(* Logix 5000 AddOnInstructionDefinition export SIKO_AG2X; software revision 18.02 *)

ADD_ON_INSTRUCTION SIKO_AG2X   (* revision 1.6, vendor SIKO GmbH *)
// SIKO DriveLine AG2X AOI
// Revision note:
// minor changes, timeout feature added
VAR_INPUT
   Cmd_OFF1 : BOOL; {visible}
   Cmd_OFF2 : BOOL; {visible}
   Cmd_OFF3 : BOOL; {visible}
   Cmd_Intermediate_stop : BOOL; {visible}
   Cmd_Start_travel_job : BOOL; {visible}
   Cmd_Acknowledge_error : BOOL; {visible}
   Cmd_Inching_mode_1 : BOOL; {visible}
   Cmd_Inching_2_Pos : BOOL; {visible}
   Cmd_Inching_2_Neg : BOOL; {visible}
   Cmd_Move_relative : BOOL; {visible}
END_VAR
VAR_IN_OUT
   DC_OUTPUT : SINT[7]; {required}
   DC_INPUT : SINT[7]; {required}
END_VAR
VAR_INPUT
   Cmd_Start_read : BOOL; {visible}
   Cmd_Start_write : BOOL; {visible}
END_VAR
VAR_IN_OUT
   GetMsg : MESSAGE; {required}
   GetMsgData : SINT[4]; {required}
   SetMsg : MESSAGE; {required}
   SetMsgData : SINT[4]; {required}
END_VAR
VAR_OUTPUT
   count_read : INT; {access Read Only, visible}
   read_error : DINT; {access Read Only, visible}
   count_write : INT; {access Read Only, visible}
   write_error : DINT; {access Read Only, visible}
END_VAR
VAR_INPUT
   Cmd_DO1 : BOOL; {visible}
END_VAR
VAR_OUTPUT
   ACTUAL_VALUE : DINT; {access Read Only, visible}
END_VAR
VAR_INPUT
   TARGET_VALUE : DINT; {visible}
   Cmd_Copy_r_to_w : BOOL; {visible}
   Cmd_BIT9 : BOOL;
   Cmd_BIT10 : BOOL;
   Cmd_BIT11 : BOOL;
   Cmd_BIT12 : BOOL;
   Cmd_BIT13 : BOOL;
   Cmd_BIT14 : BOOL;
   Cmd_BIT15 : BOOL;
END_VAR
VAR_OUTPUT
   i0513_Led_functionality_r : SINT; {access Read Only}
END_VAR
VAR_INPUT
   i0513_Led_functionality_w : SINT;
END_VAR
VAR_OUTPUT
   i0545_Si_baudrate_r : SINT; {access Read Only}
END_VAR
VAR_INPUT
   i0545_Si_baudrate_w : SINT := 1;
END_VAR
VAR_OUTPUT
   i0769_DO_1_functionality_r : SINT; {access Read Only}
END_VAR
VAR_INPUT
   i0769_DO_1_functionality_w : SINT;
END_VAR
VAR_OUTPUT
   i0770_DO_functionalities_state_r : DINT; {access Read Only}
   i0771_DO_polarity_r : SINT; {access Read Only}
END_VAR
VAR_INPUT
   i0771_DO_polarity_w : SINT;
END_VAR
VAR_OUTPUT
   i1025_DI_1_functionality_r : SINT; {access Read Only}
END_VAR
VAR_INPUT
   i1025_DI_1_functionality_w : SINT;
END_VAR
VAR_OUTPUT
   i1026_DI_2_functionality_r : SINT; {access Read Only}
END_VAR
VAR_INPUT
   i1026_DI_2_functionality_w : SINT;
END_VAR
VAR_OUTPUT
   i1027_DI_3_functionality_r : SINT; {access Read Only}
END_VAR
VAR_INPUT
   i1027_DI_3_functionality_w : SINT;
END_VAR
VAR_OUTPUT
   i1028_DI_4_functionality_r : SINT; {access Read Only}
END_VAR
VAR_INPUT
   i1028_DI_4_functionality_w : SINT;
END_VAR
VAR_OUTPUT
   i1029_DI_functionalities_state_r : DINT; {access Read Only}
   i1030_DI_polarity_r : SINT; {access Read Only}
END_VAR
VAR_INPUT
   i1030_DI_polarity_w : SINT;
END_VAR
VAR_OUTPUT
   i1537_Controller_parameter_P_r : INT; {access Read Only}
END_VAR
VAR_INPUT
   i1537_Controller_parameter_P_w : INT := 300;
END_VAR
VAR_OUTPUT
   i1538_Controller_parameter_I_r : INT; {access Read Only}
END_VAR
VAR_INPUT
   i1538_Controller_parameter_I_w : INT := 2;
END_VAR
VAR_OUTPUT
   i1539_Controller_parameter_D_r : INT; {access Read Only}
END_VAR
VAR_INPUT
   i1539_Controller_parameter_D_w : INT;
END_VAR
VAR_OUTPUT
   i1540_a_Pos_r : INT; {access Read Only}
END_VAR
VAR_INPUT
   i1540_a_Pos_w : INT := 50;
END_VAR
VAR_OUTPUT
   i1541_v_Pos_r : INT; {access Read Only}
END_VAR
VAR_INPUT
   i1541_v_Pos_w : INT := 10;
END_VAR
VAR_OUTPUT
   i1542_d_Pos_r : INT; {access Read Only}
END_VAR
VAR_INPUT
   i1542_d_Pos_w : INT := 101;
END_VAR
VAR_OUTPUT
   i1543_a_Rot_r : INT; {access Read Only}
END_VAR
VAR_INPUT
   i1543_a_Rot_w : INT := 50;
END_VAR
VAR_OUTPUT
   i1544_a_Inch_r : INT; {access Read Only}
END_VAR
VAR_INPUT
   i1544_a_Inch_w : INT := 50;
END_VAR
VAR_OUTPUT
   i1545_v_Inch_r : INT; {access Read Only}
END_VAR
VAR_INPUT
   i1545_v_Inch_w : INT := 10;
END_VAR
VAR_OUTPUT
   i1546_Pos_window_r : INT; {access Read Only}
END_VAR
VAR_INPUT
   i1546_Pos_window_w : INT := 10;
END_VAR
VAR_OUTPUT
   i1547_Gear_ratio_numerator_r : INT; {access Read Only}
END_VAR
VAR_INPUT
   i1547_Gear_ratio_numerator_w : INT := 1;
END_VAR
VAR_OUTPUT
   i1548_Gear_ratio_denominator_r : INT; {access Read Only}
END_VAR
VAR_INPUT
   i1548_Gear_ratio_denominator_w : INT := 1;
END_VAR
VAR_OUTPUT
   i1549_Spindle_pitch_r : DINT; {access Read Only}
END_VAR
VAR_INPUT
   i1549_Spindle_pitch_w : DINT;
END_VAR
VAR_OUTPUT
   i1550_Calibration_value_r : DINT; {access Read Only}
END_VAR
VAR_INPUT
   i1550_Calibration_value_w : DINT;
END_VAR
VAR_OUTPUT
   i1551_Limit_1_r : DINT; {access Read Only}
END_VAR
VAR_INPUT
   i1551_Limit_1_w : DINT := 99999;
END_VAR
VAR_OUTPUT
   i1552_Limit_2_r : DINT; {access Read Only}
END_VAR
VAR_INPUT
   i1552_Limit_2_w : DINT := -19999;
END_VAR
VAR_OUTPUT
   i1553_Delta_inch_r : DINT; {access Read Only}
END_VAR
VAR_INPUT
   i1553_Delta_inch_w : DINT := 720;
END_VAR
VAR_OUTPUT
   i1554_Sense_of_rotation_r : SINT; {access Read Only}
END_VAR
VAR_INPUT
   i1554_Sense_of_rotation_w : SINT;
END_VAR
VAR_OUTPUT
   i1555_Pos_type_r : SINT; {access Read Only}
END_VAR
VAR_INPUT
   i1555_Pos_type_w : SINT;
END_VAR
VAR_OUTPUT
   i1556_Operating_mode_r : SINT; {access Read Only}
END_VAR
VAR_INPUT
   i1556_Operating_mode_w : SINT;
END_VAR
VAR_OUTPUT
   i1557_Inching_2_stop_mode_r : SINT; {access Read Only}
END_VAR
VAR_INPUT
   i1557_Inching_2_stop_mode_w : SINT;
END_VAR
VAR_OUTPUT
   i1558_Inpos_mode_r : SINT; {access Read Only}
END_VAR
VAR_INPUT
   i1558_Inpos_mode_w : SINT;
END_VAR
VAR_OUTPUT
   i1559_Loop_length_r : INT;
END_VAR
VAR_INPUT
   i1559_Loop_length_w : INT := 360;
END_VAR
VAR_OUTPUT
   i1560_Contouring_error_limit_r : INT; {access Read Only}
END_VAR
VAR_INPUT
   i1560_Contouring_error_limit_w : INT := 400;
END_VAR
VAR_OUTPUT
   i1561_Current_limiting_r : SINT; {access Read Only}
END_VAR
VAR_INPUT
   i1561_Current_limiting_w : SINT := 110;
END_VAR
VAR_OUTPUT
   i1562_Inching_2_Offset_r : SINT; {access Read Only}
END_VAR
VAR_INPUT
   i1562_Inching_2_Offset_w : SINT := 100;
END_VAR
VAR_OUTPUT
   i1563_Inching_2_acceleration_type_r : SINT; {access Read Only}
END_VAR
VAR_INPUT
   i1563_Inching_2_acceleration_type_w : SINT;
END_VAR
VAR_OUTPUT
   i1564_Offset_r : DINT; {access Read Only}
END_VAR
VAR_INPUT
   i1564_Offset_w : DINT;
END_VAR
VAR_OUTPUT
   i2338_Pcm_pos_1_r : DINT; {access Read Only}
END_VAR
VAR_INPUT
   i2338_Pcm_pos_1_w : DINT; {access Read Only}
END_VAR
VAR_OUTPUT
   i2339_Pcm_pos_2_r : DINT; {access Read Only}
END_VAR
VAR_INPUT
   i2339_Pcm_pos_2_w : DINT; {access Read Only}
END_VAR
VAR_OUTPUT
   i2340_Pcm_pos_3_r : DINT; {access Read Only}
END_VAR
VAR_INPUT
   i2340_Pcm_pos_3_w : DINT; {access Read Only}
END_VAR
VAR_OUTPUT
   i2341_Pcm_pos_4_r : DINT; {access Read Only}
END_VAR
VAR_INPUT
   i2341_Pcm_pos_4_w : DINT; {access Read Only}
END_VAR
VAR_OUTPUT
   i2342_Pcm_pos_5_r : DINT; {access Read Only}
END_VAR
VAR_INPUT
   i2342_Pcm_pos_5_w : DINT; {access Read Only}
END_VAR
VAR_OUTPUT
   i2343_Pcm_pos_6_r : DINT; {access Read Only}
END_VAR
VAR_INPUT
   i2343_Pcm_pos_6_w : DINT; {access Read Only}
END_VAR
VAR_OUTPUT
   i2344_Pcm_pos_7_r : DINT; {access Read Only}
END_VAR
VAR_INPUT
   i2344_Pcm_pos_7_w : DINT; {access Read Only}
END_VAR
VAR_OUTPUT
   i2370_Pcm_acc_1_r : INT; {access Read Only}
END_VAR
VAR_INPUT
   i2370_Pcm_acc_1_w : INT := 50; {access Read Only}
END_VAR
VAR_OUTPUT
   i2371_Pcm_acc_2_r : INT; {access Read Only}
END_VAR
VAR_INPUT
   i2371_Pcm_acc_2_w : INT := 50; {access Read Only}
END_VAR
VAR_OUTPUT
   i2372_Pcm_acc_3_r : INT; {access Read Only}
END_VAR
VAR_INPUT
   i2372_Pcm_acc_3_w : INT := 50; {access Read Only}
END_VAR
VAR_OUTPUT
   i2373_Pcm_acc_4_r : INT; {access Read Only}
END_VAR
VAR_INPUT
   i2373_Pcm_acc_4_w : INT := 50;
END_VAR
VAR_OUTPUT
   i2374_Pcm_acc_5_r : INT; {access Read Only}
END_VAR
VAR_INPUT
   i2374_Pcm_acc_5_w : INT := 50;
END_VAR
VAR_OUTPUT
   i2375_Pcm_acc_6_r : INT; {access Read Only}
END_VAR
VAR_INPUT
   i2375_Pcm_acc_6_w : INT := 50;
END_VAR
VAR_OUTPUT
   i2376_Pcm_acc_7_r : INT; {access Read Only}
END_VAR
VAR_INPUT
   i2376_Pcm_acc_7_w : INT := 50;
END_VAR
VAR_OUTPUT
   i2402_Pcm_vel_1_r : INT; {access Read Only}
END_VAR
VAR_INPUT
   i2402_Pcm_vel_1_w : INT := 10;
END_VAR
VAR_OUTPUT
   i2403_Pcm_vel_2_r : INT; {access Read Only}
END_VAR
VAR_INPUT
   i2403_Pcm_vel_2_w : INT := 10;
END_VAR
VAR_OUTPUT
   i2404_Pcm_vel_3_r : INT; {access Read Only}
END_VAR
VAR_INPUT
   i2404_Pcm_vel_3_w : INT := 10;
END_VAR
VAR_OUTPUT
   i2405_Pcm_vel_4_r : INT; {access Read Only}
END_VAR
VAR_INPUT
   i2405_Pcm_vel_4_w : INT := 10;
END_VAR
VAR_OUTPUT
   i2406_Pcm_vel_5_r : INT; {access Read Only}
END_VAR
VAR_INPUT
   i2406_Pcm_vel_5_w : INT := 10;
END_VAR
VAR_OUTPUT
   i2407_Pcm_vel_6_r : INT; {access Read Only}
END_VAR
VAR_INPUT
   i2407_Pcm_vel_6_w : INT := 10;
END_VAR
VAR_OUTPUT
   i2408_Pcm_vel_7_r : INT; {access Read Only}
END_VAR
VAR_INPUT
   i2408_Pcm_vel_7_w : INT := 10;
END_VAR
VAR_OUTPUT
   i2434_Pcm_dec_1_r : INT; {access Read Only}
END_VAR
VAR_INPUT
   i2434_Pcm_dec_1_w : INT := 101;
END_VAR
VAR_OUTPUT
   i2435_Pcm_dec_2_r : INT; {access Read Only}
END_VAR
VAR_INPUT
   i2435_Pcm_dec_2_w : INT := 101;
END_VAR
VAR_OUTPUT
   i2436_Pcm_dec_3_r : INT; {access Read Only}
END_VAR
VAR_INPUT
   i2436_Pcm_dec_3_w : INT := 101;
END_VAR
VAR_OUTPUT
   i2437_Pcm_dec_4_r : INT; {access Read Only}
END_VAR
VAR_INPUT
   i2437_Pcm_dec_4_w : INT := 101;
END_VAR
VAR_OUTPUT
   i2438_Pcm_dec_5_r : INT; {access Read Only}
END_VAR
VAR_INPUT
   i2438_Pcm_dec_5_w : INT := 101;
END_VAR
VAR_OUTPUT
   i2439_Pcm_dec_6_r : INT; {access Read Only}
END_VAR
VAR_INPUT
   i2439_Pcm_dec_6_w : INT := 101;
END_VAR
VAR_OUTPUT
   i2440_Pcm_dec_7_r : INT; {access Read Only}
END_VAR
VAR_INPUT
   i2440_Pcm_dec_7_w : INT := 101;
END_VAR
VAR_OUTPUT
   i2561_Output_stage_temperature_r : INT; {access Read Only}
   i2562_Voltage_of_control_r : INT; {access Read Only}
   i2563_Voltage_of_output_power_stage_r : INT; {access Read Only}
   i2564_Voltage_of_battery_r : INT; {access Read Only}
   i2565_Motor_Current_r : INT; {access Read Only}
   i2566_Actual_position_r : DINT; {access Read Only}
   i2567_Actual_rotational_speed_r : INT; {access Read Only}
   i2568_Serial_number_r : DINT; {access Read Only}
   i2569_Production_date_r : DINT; {access Read Only}
   i2570_Sw_motor_controller_r : DINT; {access Read Only}
   i2571_Gear_reduction_r : INT; {access Read Only}
   i2572_System_status_word_r : INT;
   i2573_Encoder_resolution_r : INT; {access Read Only}
   i2574_Device_id_r : SINT; {access Read Only}
   i2817_Number_of_errors_r : SINT; {access Read Only}
   i2818_Error_nbr_1_r : SINT; {access Read Only}
   i2819_Error_nbr_2_r : SINT; {access Read Only}
   i2820_Error_nbr_3_r : SINT; {access Read Only}
   i2821_Error_nbr_4_r : SINT; {access Read Only}
   i2822_Error_nbr_5_r : SINT; {access Read Only}
   i2823_Error_nbr_6_r : SINT; {access Read Only}
   i2824_Error_nbr_7_r : SINT; {access Read Only}
   i2825_Error_nbr_8_r : SINT; {access Read Only}
   i2826_Error_nbr_9_r : SINT; {access Read Only}
   i2827_Error_nbr_10_r : SINT; {access Read Only}
   i3073_S_command_r : SINT; {access Read Only}
END_VAR
VAR_INPUT
   i3073_S_command_w : SINT;
END_VAR
VAR_OUTPUT
   Sts_BIT13 : BOOL; {access Read Only}
   Sts_BIT14 : BOOL; {access Read Only}
   Sts_BIT15 : BOOL; {access Read Only}
   Sts_Supply : BOOL; {access Read Only, visible}
   Sts_Readiness_to_travel : BOOL; {access Read Only, visible}
   Sts_Upper_limit : BOOL; {access Read Only, visible}
   Sts_Lower_limit : BOOL; {access Read Only, visible}
   Sts_Actuator_travels_stands : BOOL; {access Read Only, visible}
   Sts_InPos : BOOL; {access Read Only, visible}
   Sts_Active_travel_job : BOOL; {access Read Only, visible}
   Sts_Error : BOOL; {access Read Only, visible}
   Sts_Operation_enabled : BOOL; {access Read Only, visible}
   Sts_Switch_lock : BOOL; {access Read Only, visible}
   Sts_Travel_job_acknowledge : BOOL; {access Read Only, visible}
   Sts_Battery_warning : BOOL; {access Read Only, visible}
   Sts_Current_limiting : BOOL; {access Read Only, visible}
   Sts_DI1 : BOOL; {access Read Only, visible}
   Sts_DI2 : BOOL; {access Read Only, visible}
   Sts_DI3 : BOOL; {access Read Only, visible}
   Sts_DI4 : BOOL; {access Read Only, visible}
   Sts_Done : BOOL; {access Read Only, visible}
   Sts_Busy : BOOL; {access Read Only, visible}
   Sts_General_error : BOOL; {access Read Only, visible}
END_VAR
VAR_INPUT
   Timeout : DINT := 5000; {visible}
END_VAR
VAR
   BTDT_01 : FBD_BIT_FIELD_DISTRIBUTE := (Length := 1); {access None}
   BTDT_02 : FBD_BIT_FIELD_DISTRIBUTE := (Length := 1); {access None}
   DC_INPUT_BUF : SINT[7]; {access None}
   DC_OUTPUT_BUF : SINT[7]; {access None}
   GetMsgStep : INT; {access None}
   SetMsgStep : INT; {access None}
   LD_OUT : DINT; {access None}
   OSR_copy : BOOL; {access None}
   OSR_read : BOOL; {access None}
   OSR_write : BOOL; {access None}
   SetMsgFlags : INT; {access None}
   GetMsgFlags : INT; {access None}
   COUNTER_WRITE : INT; {access None}
   COUNTER_READ : INT; {access None}
   COUNTER_COPY : INT; {access None}
   tTOutWrite : FBD_TIMER; {access None}
   tTOutRead : FBD_TIMER; {access None}
END_VAR

ROUTINE Logic   (* structured text *)
   ///////////////////////////////////////////////////////////////////////////////////////////////
   // Name:	SIKO_AG2X
   ///////////////////////////////////////////////////////////////////////////////////////////////
   // Version history
   ///////////////////////////////////////////////////////////////////////////////////////////////
   // Date        | Version  | created under          	| Author    		| Remark
   // dd.mm.yyyy  | 		  |							|					|
   // -----------------------------------------------------------------------------------
   // 17.06.2014  | 1.0.0    | V20.01.00 (CPR 9 SR 5) 	| SIKO GmbH / hof 	| first release
   // 04.07.2014  | 1.1.0	  | V20.01.00 (CPR 9 SR 5)  | SIKO GmbH / hof 	| synchronous access
   // 06.10.2014  | 1.2.0    | V20.01.00 (CPR 9 SR 5)  | SIKO GmbH / hof 	| minor changes
   // 04.02.2015  | 1.3.0    | V20.01.00 (CPR 9 SR 5)  | SIKO GmbH / hof   | signature protection
   // 05.03.2015  | 1.4.0    | V20.01.00 (CPR 9 SR 5)  | SIKO GmbH / hof   | cycle time optimization
   // 02.06.2015  | 1.5.0    | V20.01.00 (CPR 9 SR 5)  | SIKO GmbH / hof   | memory optimization
   // 12.08.2015  | 1.6.0	  | V20.01.00 (CPR 9 SR 5)  | SIKO GmbH / hof   | minor changes, timeout feature added
    ///////////////////////////////////////////////////////////////////////////////////////////////
   
   ///////////////////////////////////////////////////////////////////////////////////////////////
   // Init at first scan
   //
   IF s:fs THEN
   	Sts_Done := 0;
   	Sts_Busy := 0;
   	Sts_General_error := 0;
   	read_error := 0;
   	write_error := 0;
   	count_read := 0;
   	count_write := 0;
   	COUNTER_WRITE := 0;
   	COUNTER_READ := 0;
   	COUNTER_COPY := 0;
   	OSR_read := 0;
   	OSR_write := 0;
   	OSR_copy := 0;
       GetMsgStep := 0;
   	SetMsgStep := 0;
   END_IF;
   
   ///////////////////////////////////////////////////////////////////////////////////////////////
   // read inputs synchonous
   CPS(DC_INPUT[0],DC_INPUT_BUF[0],7);
   
   ///////////////////////////////////////////////////////////////////////////////////////////////
   // target value
   // DINT TO SINT[4]
   
   COP(TARGET_VALUE,DC_OUTPUT_BUF[2],4);
   
   ///////////////////////////////////////////////////////////////////////////////////////////////
   
   ///////////////////////////////////////////////////////////////////////////////////////////////
   // control word
   //
   
   DC_OUTPUT_BUF[0].0 := Cmd_OFF1;
   DC_OUTPUT_BUF[0].1 := Cmd_OFF2;
   DC_OUTPUT_BUF[0].2 := Cmd_OFF3;
   DC_OUTPUT_BUF[0].3 := Cmd_Intermediate_stop;
   DC_OUTPUT_BUF[0].4 := Cmd_Start_travel_job;
   DC_OUTPUT_BUF[0].5 := Cmd_Acknowledge_error;
   DC_OUTPUT_BUF[0].6 := Cmd_Inching_mode_1;
   DC_OUTPUT_BUF[0].7 := Cmd_Inching_2_Pos;
   DC_OUTPUT_BUF[1].0 := Cmd_Inching_2_Neg;
   DC_OUTPUT_BUF[1].1 := Cmd_BIT9;
   DC_OUTPUT_BUF[1].2 := Cmd_Move_relative;
   DC_OUTPUT_BUF[1].3 := Cmd_BIT11;
   DC_OUTPUT_BUF[1].4 := Cmd_BIT12;
   DC_OUTPUT_BUF[1].5 := Cmd_BIT13;
   DC_OUTPUT_BUF[1].6 := Cmd_BIT14;
   DC_OUTPUT_BUF[1].7 := Cmd_BIT15;
   
   ///////////////////////////////////////////////////////////////////////////////////////////////
   // digital outputs
   //
   DC_OUTPUT_BUF[6].0 := Cmd_DO1;
   
   ///////////////////////////////////////////////////////////////////////////////////////////////
   // start read
   //
   IF Cmd_Start_read AND (COUNTER_COPY = 0) AND (COUNTER_READ = 0) AND (COUNTER_WRITE = 0) AND NOT OSR_read
   THEN
   	Sts_Done := 0;
   	Sts_Busy := 1;
   	Sts_General_error := 0;
   	read_error := 0;
   	write_error := 0;
   	count_read := 0;
   	count_write := 0;
   	COUNTER_WRITE := 0;
   	COUNTER_READ := 1;
   	OSR_read := 1;
   END_IF;
   
   IF NOT Cmd_Start_read and OSR_read
   THEN
   	OSR_read := 0;
   END_IF;
   
   ///////////////////////////////////////////////////////////////////////////////////////////////
   // start write
   //
   
   IF Cmd_Start_write AND (COUNTER_COPY = 0) AND (COUNTER_READ = 0) AND (COUNTER_WRITE = 0) AND NOT OSR_write
   THEN
   	Sts_Done := 0;
   	Sts_Busy := 1;
   	Sts_General_error := 0;
   	read_error := 0;
   	write_error := 0;
   	count_read := 0;
   	count_write := 0;
   	COUNTER_WRITE := 1;
   	COUNTER_READ := 0;
   	OSR_write := 1;
   END_IF;
   
   IF NOT Cmd_Start_write and OSR_write
   THEN
   	OSR_write := 0;
   END_IF;
   
   ///////////////////////////////////////////////////////////////////////////////////////////////
   // copy read to write parameters
   //
   
   IF Cmd_Copy_r_to_w AND (COUNTER_COPY = 0) AND (COUNTER_READ = 0) AND (COUNTER_WRITE = 0) AND NOT OSR_copy
   THEN
   	Sts_Done := 0;
   	Sts_Busy := 1;
   	Sts_General_error := 0;
   	read_error := 0;
   	write_error := 0;
   	count_read := 0;
   	count_write := 0;
   	OSR_copy := 1;
   	COUNTER_COPY := 1;
   END_IF;
   
   IF NOT Cmd_Copy_r_to_w and OSR_copy
   THEN
   	OSR_copy := 0;
   END_IF;
   
   ///////////////////////////////////////////////////////////////////////////////////////////////
   // Timeout read function
   //
   IF GetMsgStep <> 0 THEN
   	tTOutRead.TimerEnable:= 1;
   ELSE
   	tTOutRead.TimerEnable:= 0;
   END_IF;
   tTOutRead.PRE:= Timeout;
   TONR(tTOutRead);
   
   IF tTOutRead.DN THEN
   	// set status bits
   	Sts_Done := 0;
   	Sts_Busy := 0;
   	Sts_General_error := 1;
   
     	GetMsgStep := 0;
   	count_read := COUNTER_READ;
   	COUNTER_READ := 0;
   
   	// copy error code to read_error
   	BTDT_01.Source := 16#F001; // Timeout error
   	BTDT_01.SourceBit := 0;
   	BTDT_01.Length := 16;
   	BTDT_01.DestBit := 0;
   	BTDT_01.Target := read_error;
   	BTDT(BTDT_01);
   	read_error := BTDT_01.Dest;
   
   	// copy extended error code to read_error
   	BTDT_01.Source := 0;
   	BTDT_01.SourceBit := 0;
   	BTDT_01.Length := 16;
   	BTDT_01.DestBit := 16;
   	BTDT_01.Target := read_error;
   	BTDT(BTDT_01);
   	read_error := BTDT_01.Dest;
   END_IF;
   
   ///////////////////////////////////////////////////////////////////////////////////////////////
   // Timeout write function
   //
   IF SetMsgStep <> 0 THEN
   	tTOutWrite.TimerEnable:= 1;
   ELSE
   	tTOutWrite.TimerEnable:= 0;
   END_IF;
   tTOutWrite.PRE:= Timeout;
   TONR(tTOutWrite);
   
   IF tTOutWrite.DN THEN
   	// set status bits
   	Sts_Done := 0;
   	Sts_Busy := 0;
   	Sts_General_error := 1;
   
   	SetMsgStep := 0;
   	count_write := COUNTER_WRITE;
   	COUNTER_WRITE := 0;
   	write_error := 0;
   
   	// copy error code to write_error
   	BTDT_02.Source := 16#F001; // Timeout error
   	BTDT_02.SourceBit := 0;
   	BTDT_02.Length := 16;
   	BTDT_02.DestBit := 0;
   	BTDT_02.Target := write_error;
   	BTDT(BTDT_02);
   	write_error := BTDT_02.Dest;
   
   	// copy extended error code to write_error
   	BTDT_02.Source := 0;
   	BTDT_02.SourceBit := 0;
   	BTDT_02.Length := 16;
   	BTDT_02.DestBit := 16;
   	BTDT_02.Target := write_error;
   	BTDT(BTDT_02);
   	write_error := BTDT_02.Dest;
   END_IF;
   
   ///////////////////////////////////////////////////////////////////////////////////////////////
   // handle read instruction
   //
   
   IF (GetMsgStep = 0) AND (COUNTER_READ > 0)
   THEN
   
   	//--> common settings for read requests
   	GetMsg.REQ_LEN := 0;
   	GetMsg.Class := 16#A2;
   	GetMsg.Attribute := 5;
   	//<--
   
   	CASE COUNTER_READ OF // read request
   	1:  // LED Functionality
   		GetMsg.Instance := 513;
   	2:  // Service Interface Baud Rate
   		GetMsg.Instance := 545;
   	3:  // Digital Output 1 Functionality
   		GetMsg.Instance := 769;
   	4:  // Digital Output Functionalities State
   		GetMsg.Instance := 770;
   	5:  // Digital Outputs Polarity
   		GetMsg.Instance := 771;
   	6:  // Digital Input 1 Functionality
   		GetMsg.Instance := 1025;
   	7:  // Digital Input 2 Functionality
   		GetMsg.Instance := 1026;
   	8:  // Digital Input 3 Functionality
   		GetMsg.Instance := 1027;
   	9:  // Digital Input 4 Functionality
   		GetMsg.Instance := 1028;
   	10:  // Digital Input Functionalities State
   		GetMsg.Instance := 1029;
   	11:  // Digital Inputs Polarity
   		GetMsg.Instance := 1030;
   	12:  // Controller Parameter P
   		GetMsg.Instance := 1537;
   	13:  // Controller Parameter I
   		GetMsg.Instance := 1538;
   	14:  // Controller Parameter D
   		GetMsg.Instance := 1539;
   	15:  // A-Pos
   		GetMsg.Instance := 1540;
   	16:  // V-Pos
   		GetMsg.Instance := 1541;
   	17:  // D-Pos
   		GetMsg.Instance := 1542;
   	18:  // A-Rot
   		GetMsg.Instance := 1543;
   	19:  // A-Inch
   		GetMsg.Instance := 1544;
   	20:  // V-Inch
   		GetMsg.Instance := 1545;
   	21:  // Pos Window
   		GetMsg.Instance := 1546;
   	22:  // Gear Ratio Numerator
   		GetMsg.Instance := 1547;
   	23:  // Gear Ratio Denominator
   		GetMsg.Instance := 1548;
   	24:  // Spindle Pitch
   		GetMsg.Instance := 1549;
   	25:  // Calibration Value
   		GetMsg.Instance := 1550;
   	26:  // Software Limit 1
   		GetMsg.Instance := 1551;
   	27:  // Software Limit 2
   		GetMsg.Instance := 1552;
   	28:  // Delta Inch
   		GetMsg.Instance := 1553;
   	29:  // Sense of Rotation
   		GetMsg.Instance := 1554;
   	30:  // Pos Type
   		GetMsg.Instance := 1555;
   	31:  // Operating Mode
   		GetMsg.Instance := 1556;
   	32:  // Inching 2 Stop Mode
   		GetMsg.Instance := 1557;
   	33:  // Inpos Mode
   		GetMsg.Instance := 1558;
   	34:  // Loop Length
   		GetMsg.Instance := 1559;
   	35:  // Contouring Error Limit
   		GetMsg.Instance := 1560;
   	36:  // Current Limiting
   		GetMsg.Instance := 1561;
   	37:  // Inching 2 Offset
   		GetMsg.Instance := 1562;
   	38:  // Inching 2 Acceleration Type
   		GetMsg.Instance := 1563;
   	39:  // Offset Value
   		GetMsg.Instance := 1564;
   	40:  // PCM Position 1
   		GetMsg.Instance := 2338;
   	41:  // PCM Position 2
   		GetMsg.Instance := 2339;
   	42:  // PCM Position 3
   		GetMsg.Instance := 2340;
   	43:  // PCM Position 4
   		GetMsg.Instance := 2341;
   	44:  // PCM Position 5
   		GetMsg.Instance := 2342;
   	45:  // PCM Position 6
   		GetMsg.Instance := 2343;
   	46:  // PCM Position 7
   		GetMsg.Instance := 2344;
   	47:  // PCM Acceleration 1
   		GetMsg.Instance := 2370;
   	48:  // PCM Acceleration 2
   		GetMsg.Instance := 2371;
   	49:  // PCM Acceleration 3
   		GetMsg.Instance := 2372;
   	50:  // PCM Acceleration 4
   		GetMsg.Instance := 2373;
   	51:  // PCM Acceleration 5
   		GetMsg.Instance := 2374;
   	52:  // PCM Acceleration 6
   		GetMsg.Instance := 2375;
   	53:  // PCM Acceleration 7
   		GetMsg.Instance := 2376;
   	54:  // PCM Velocitiy 1
   		GetMsg.Instance := 2402;
   	55:  // PCM Velocitiy 2
   		GetMsg.Instance := 2403;
   	56:  // PCM Velocitiy 3
   		GetMsg.Instance := 2404;
   	57:  // PCM Velocitiy 4
   		GetMsg.Instance := 2405;
   	58:  // PCM Velocitiy 5
   		GetMsg.Instance := 2406;
   	59:  // PCM Velocitiy 6
   		GetMsg.Instance := 2407;
   	60:  // PCM Velocitiy 7
   		GetMsg.Instance := 2408;
   	61:  // PCM Deceleration 1
   		GetMsg.Instance := 2434;
   	62:  // PCM Deceleration 2
   		GetMsg.Instance := 2435;
   	63:  // PCM Deceleration 3
   		GetMsg.Instance := 2436;
   	64:  // PCM Deceleration 4
   		GetMsg.Instance := 2437;
   	65:  // PCM Deceleration 5
   		GetMsg.Instance := 2438;
   	66:  // PCM Deceleration 6
   		GetMsg.Instance := 2439;
   	67:  // PCM Deceleration 7
   		GetMsg.Instance := 2440;
   	68:  // Output Stage Temperature
   		GetMsg.Instance := 2561;
   	69:  // Voltage of Control
   		GetMsg.Instance := 2562;
   	70:  // Voltage of Output Stage
   		GetMsg.Instance := 2563;
   	71:  // Voltage of Battery
   		GetMsg.Instance := 2564;
   	72:  // Motor Current
   		GetMsg.Instance := 2565;
   	73:  // Actual Position
   		GetMsg.Instance := 2566;
   	74:  // Actual Rotational Speed
   		GetMsg.Instance := 2567;
   	75:  // Serial Number
   		GetMsg.Instance := 2568;
   	76:  // Production Date
   		GetMsg.Instance := 2569;
   	77:  // SW Motor Controller
   		GetMsg.Instance := 2570;
   	78:  // Gear Reduction
   		GetMsg.Instance := 2571;
   	79:  // System Status Word
   		GetMsg.Instance := 2572;
   	80:  // Encoder Resolution
   		GetMsg.Instance := 2573;
   	81:  // Device ID
   		GetMsg.Instance := 2574;
   	82:  // Number of Errors
   		GetMsg.Instance := 2817;
   	83:  // Error Number 1
   		GetMsg.Instance := 2818;
   	84:  // Error Number 2
   		GetMsg.Instance := 2819;
   	85:  // Error Number 3
   		GetMsg.Instance := 2820;
   	86:  // Error Number 4
   		GetMsg.Instance := 2821;
   	87:  // Error Number 5
   		GetMsg.Instance := 2822;
   	88:  // Error Number 6
   		GetMsg.Instance := 2823;
   	89:  // Error Number 7
   		GetMsg.Instance := 2824;
   	90:  // Error Number 8
   		GetMsg.Instance := 2825;
   	91:  // Error Number 9
   		GetMsg.Instance := 2826;
   	92:  // Error Number 10
   		GetMsg.Instance := 2827;
   	END_CASE;
   
   	// clear input buffer
   	GetMsgData[0] := 0;
   	GetMsgData[1] := 0;
   	GetMsgData[2] := 0;
   	GetMsgData[3] := 0;
   
   	// send message request
   	GetMsgStep := 1;
   END_IF;
   
   // send message
   IF GetMsgStep = 1 THEN
   	MSG(GetMsg);
   	GetMsgStep := 2;
   END_IF;
   
   // create local copy of GetMsg.FLAGS
   GetMsgFlags := GetMsg.FLAGS;
   
   IF(GetMsgStep = 2) AND (GetMsgFlags.4) THEN
   // .ER bit set = transfer failed
     	GetMsgStep := 0;
   	count_read := COUNTER_READ;
   	read_error := 0;
   
   	// copy error code to read_error
   	BTDT_01.Source := GetMsg.ERR;
   	BTDT_01.SourceBit := 0;
   	BTDT_01.Length := 16;
   	BTDT_01.DestBit := 0;
   	BTDT_01.Target := read_error;
   	BTDT(BTDT_01);
   	read_error := BTDT_01.Dest;
   
   	// copy extended error code to read_error
   	BTDT_01.Source := GetMsg.EXERR;
   	BTDT_01.SourceBit := 0;
   	BTDT_01.Length := 16;
   	BTDT_01.DestBit := 16;
   	BTDT_01.Target := read_error;
   	BTDT(BTDT_01);
   	read_error := BTDT_01.Dest;
   
   	// set status bits
   	Sts_Done := 0;
   	Sts_Busy := 0;
   	Sts_General_error := 1;
   
   	COUNTER_READ := 0;
   ELSIF (GetMsgStep = 2) AND (GetMsgFlags.5) THEN
   // .DN bit set = transfer ok
   	GetMsgStep := 0;
   	// output only when transfer failed
   	count_read := 0;
   	read_error := 0;
   
   	// use of COP command to avoid artihmetic overflow
   
   	CASE COUNTER_READ OF // read response
   	1:
   		COP(GetMsgData[0],i0513_Led_functionality_r,1);
   	2:
   		COP(GetMsgData[0],i0545_Si_baudrate_r,1);
   	3:
   		COP(GetMsgData[0],i0769_DO_1_functionality_r,1);
   	4:
   		COP(GetMsgData[0],i0770_DO_functionalities_state_r,1);
   	5:
   		COP(GetMsgData[0],i0771_DO_polarity_r,1);
   	6:
   		COP(GetMsgData[0],i1025_DI_1_functionality_r,1);
   	7:
   		COP(GetMsgData[0],i1026_DI_2_functionality_r,1);
   	8:
   		COP(GetMsgData[0],i1027_DI_3_functionality_r,1);
   	9:
   		COP(GetMsgData[0],i1028_DI_4_functionality_r,1);
   	10:
   		COP(GetMsgData[0],i1029_DI_functionalities_state_r,1);
   	11:
   		COP(GetMsgData[0],i1030_DI_polarity_r,1);
   	12:
   		COP(GetMsgData[0],i1537_Controller_parameter_P_r,1);
   	13:
   		COP(GetMsgData[0],i1538_Controller_parameter_I_r,1);
   	14:
   		COP(GetMsgData[0],i1539_Controller_parameter_D_r,1);
   	15:
   		COP(GetMsgData[0],i1540_a_Pos_r,1);
   	16:
   		COP(GetMsgData[0],i1541_v_Pos_r,1);
   	17:
   		COP(GetMsgData[0],i1542_d_Pos_r,1);
   	18:
   		COP(GetMsgData[0],i1543_a_Rot_r,1);
   	19:
   		COP(GetMsgData[0],i1544_a_Inch_r,1);
   	20:
   		COP(GetMsgData[0],i1545_v_Inch_r,1);
   	21:
   		COP(GetMsgData[0],i1546_Pos_window_r,1);
   	22:
   		COP(GetMsgData[0],i1547_Gear_ratio_numerator_r,1);
   	23:
   		COP(GetMsgData[0],i1548_Gear_ratio_denominator_r,1);
   	24:
   		COP(GetMsgData[0],i1549_Spindle_pitch_r,1);
   	25:
   		COP(GetMsgData[0],i1550_Calibration_value_r,1);
   	26:
   		COP(GetMsgData[0],i1551_Limit_1_r,1);
   	27:
   		COP(GetMsgData[0],i1552_Limit_2_r,1);
   	28:
   		COP(GetMsgData[0],i1553_Delta_inch_r,1);
   	29:
   		COP(GetMsgData[0],i1554_Sense_of_rotation_r,1);
   	30:
   		COP(GetMsgData[0],i1555_Pos_type_r,1);
   	31:
   		COP(GetMsgData[0],i1556_Operating_mode_r,1);
   	32:
   		COP(GetMsgData[0],i1557_Inching_2_stop_mode_r,1);
   	33:
   		COP(GetMsgData[0],i1558_Inpos_mode_r,1);
   	34:
   		COP(GetMsgData[0],i1559_Loop_length_r,1);
   	35:
   		COP(GetMsgData[0],i1560_Contouring_error_limit_r,1);
   	36:
   		COP(GetMsgData[0],i1561_Current_limiting_r,1);
   	37:
   		COP(GetMsgData[0],i1562_Inching_2_Offset_r,1);
   	38:
   		COP(GetMsgData[0],i1563_Inching_2_acceleration_type_r,1);
   	39:
   		COP(GetMsgData[0],i1564_Offset_r,1);
   	40:
   		COP(GetMsgData[0],i2338_Pcm_pos_1_r,1);
   	41:
   		COP(GetMsgData[0],i2339_Pcm_pos_2_r,1);
   	42:
   		COP(GetMsgData[0],i2340_Pcm_pos_3_r,1);
   	43:
   		COP(GetMsgData[0],i2341_Pcm_pos_4_r,1);
   	44:
   		COP(GetMsgData[0],i2342_Pcm_pos_5_r,1);
   	45:
   		COP(GetMsgData[0],i2343_Pcm_pos_6_r,1);
   	46:
   		COP(GetMsgData[0],i2344_Pcm_pos_7_r,1);
   	47:
   		COP(GetMsgData[0],i2370_Pcm_acc_1_r,1);
   	48:
   		COP(GetMsgData[0],i2371_Pcm_acc_2_r,1);
   	49:
   		COP(GetMsgData[0],i2372_Pcm_acc_3_r,1);
   	50:
   		COP(GetMsgData[0],i2373_Pcm_acc_4_r,1);
   	51:
   		COP(GetMsgData[0],i2374_Pcm_acc_5_r,1);
   	52:
   		COP(GetMsgData[0],i2375_Pcm_acc_6_r,1);
   	53:
   		COP(GetMsgData[0],i2376_Pcm_acc_7_r,1);
   	54:
   		COP(GetMsgData[0],i2402_Pcm_vel_1_r,1);
   	55:
   		COP(GetMsgData[0],i2403_Pcm_vel_2_r,1);
   	56:
   		COP(GetMsgData[0],i2404_Pcm_vel_3_r,1);
   	57:
   		COP(GetMsgData[0],i2405_Pcm_vel_4_r,1);
   	58:
   		COP(GetMsgData[0],i2406_Pcm_vel_5_r,1);
   	59:
   		COP(GetMsgData[0],i2407_Pcm_vel_6_r,1);
   	60:
   		COP(GetMsgData[0],i2408_Pcm_vel_7_r,1);
   	61:
   		COP(GetMsgData[0],i2434_Pcm_dec_1_r,1);
   	62:
   		COP(GetMsgData[0],i2435_Pcm_dec_2_r,1);
   	63:
   		COP(GetMsgData[0],i2436_Pcm_dec_3_r,1);
   	64:
   		COP(GetMsgData[0],i2437_Pcm_dec_4_r,1);
   	65:
   		COP(GetMsgData[0],i2438_Pcm_dec_5_r,1);
   	66:
   		COP(GetMsgData[0],i2439_Pcm_dec_6_r,1);
   	67:
   		COP(GetMsgData[0],i2440_Pcm_dec_7_r,1);
   	68:
   		COP(GetMsgData[0],i2561_Output_stage_temperature_r,1);
   	69:
   		COP(GetMsgData[0],i2562_Voltage_of_control_r,1);
   	70:
   		COP(GetMsgData[0],i2563_Voltage_of_output_power_stage_r,1);
   	71:
   		COP(GetMsgData[0],i2564_Voltage_of_battery_r,1);
   	72:
   		COP(GetMsgData[0],i2565_Motor_Current_r,1);
   	73:
   		COP(GetMsgData[0],i2566_Actual_position_r,1);
   	74:
   		COP(GetMsgData[0],i2567_Actual_rotational_speed_r,1);
   	75:
   		COP(GetMsgData[0],i2568_Serial_number_r,1);
   	76:
   		COP(GetMsgData[0],i2569_Production_date_r,1);
   	77:
   		COP(GetMsgData[0],i2570_Sw_motor_controller_r,1);
   	78:
   		COP(GetMsgData[0],i2571_Gear_reduction_r,1);
   	79:
   		COP(GetMsgData[0],i2572_System_status_word_r,1);
   	80:
   		COP(GetMsgData[0],i2573_Encoder_resolution_r,1);
   	81:
   		COP(GetMsgData[0],i2574_Device_id_r,1);
   	82:
   		COP(GetMsgData[0],i2817_Number_of_errors_r,1);
   	83:
   		COP(GetMsgData[0],i2818_Error_nbr_1_r,1);
   	84:
   		COP(GetMsgData[0],i2819_Error_nbr_2_r,1);
   	85:
   		COP(GetMsgData[0],i2820_Error_nbr_3_r,1);
   	86:
   		COP(GetMsgData[0],i2821_Error_nbr_4_r,1);
   	87:
   		COP(GetMsgData[0],i2822_Error_nbr_5_r,1);
   	88:
   		COP(GetMsgData[0],i2823_Error_nbr_6_r,1);
   	89:
   		COP(GetMsgData[0],i2824_Error_nbr_7_r,1);
   	90:
   		COP(GetMsgData[0],i2825_Error_nbr_8_r,1);
   	91:
   		COP(GetMsgData[0],i2826_Error_nbr_9_r,1);
   	92:
   		COP(GetMsgData[0],i2827_Error_nbr_10_r,1);
   	END_CASE;
   
   	COUNTER_READ := COUNTER_READ + 1;
   	count_read := COUNTER_READ;
   END_IF;
   
   IF (COUNTER_READ > 92)
   THEN
   	COUNTER_READ := 0;
   	count_read := COUNTER_READ;
   
   	// set status bits
   	Sts_Done := 1;
   	Sts_Busy := 0;
   	Sts_General_error := 0;
   
   END_IF;
   
   ///////////////////////////////////////////////////////////////////////////////////////////////
   // handle write instruction
   //
   
   IF (SetMsgStep = 0) AND (COUNTER_WRITE > 0)
   THEN
   
   	//--> common settings for write requests
   	SetMsg.Class := 16#A2;
   	SetMsg.Attribute := 5;
   	//<--
   
   	CASE COUNTER_WRITE OF // write request
   	1:
   		IF i0513_Led_functionality_w <> i0513_Led_functionality_r
   		THEN
   			LD_OUT := i0513_Led_functionality_w;
   			SetMsg.REQ_LEN := 1;
   			SetMsg.Instance := 513;
   			SetMsgStep := 1;
   		ELSE
   			COUNTER_WRITE := COUNTER_WRITE + 1;
   		END_IF;
   	2:
   		IF i0545_Si_baudrate_w <> i0545_Si_baudrate_r
   		THEN
   			LD_OUT := i0545_Si_baudrate_w;
   			SetMsg.REQ_LEN := 1;
   			SetMsg.Instance := 545;
   			SetMsgStep := 1;
   		ELSE
   			COUNTER_WRITE := COUNTER_WRITE + 1;
   		END_IF;
   	3:
   		IF i0769_DO_1_functionality_w <> i0769_DO_1_functionality_r
   		THEN
   			LD_OUT := i0769_DO_1_functionality_w;
   			SetMsg.REQ_LEN := 1;
   			SetMsg.Instance := 769;
   			SetMsgStep := 1;
   		ELSE
   			COUNTER_WRITE := COUNTER_WRITE + 1;
   		END_IF;
   	4:
   		IF i0771_DO_polarity_w <> i0771_DO_polarity_r
   		THEN
   			LD_OUT := i0771_DO_polarity_w;
   			SetMsg.REQ_LEN := 1;
   			SetMsg.Instance := 771;
   			SetMsgStep := 1;
   		ELSE
   			COUNTER_WRITE := COUNTER_WRITE + 1;
   		END_IF;
   	5:
   		IF i1025_DI_1_functionality_w <> i1025_DI_1_functionality_r
   		THEN
   			LD_OUT := i1025_DI_1_functionality_w;
   			SetMsg.REQ_LEN := 1;
   			SetMsg.Instance := 1025;
   			SetMsgStep := 1;
   		ELSE
   			COUNTER_WRITE := COUNTER_WRITE + 1;
   		END_IF;
   	6:
   		IF i1026_DI_2_functionality_w <> i1026_DI_2_functionality_r
   		THEN
   			LD_OUT := i1026_DI_2_functionality_w;
   			SetMsg.REQ_LEN := 1;
   			SetMsg.Instance := 1026;
   			SetMsgStep := 1;
   		ELSE
   			COUNTER_WRITE := COUNTER_WRITE + 1;
   		END_IF;
   	7:
   		IF i1027_DI_3_functionality_w <> i1027_DI_3_functionality_r
   		THEN
   			LD_OUT := i1027_DI_3_functionality_w;
   			SetMsg.REQ_LEN := 1;
   			SetMsg.Instance := 1027;
   			SetMsgStep := 1;
   		ELSE
   			COUNTER_WRITE := COUNTER_WRITE + 1;
   		END_IF;
   	8:
   		IF i1028_DI_4_functionality_w <> i1028_DI_4_functionality_r
   		THEN
   			LD_OUT := i1028_DI_4_functionality_w;
   			SetMsg.REQ_LEN := 1;
   			SetMsg.Instance := 1028;
   			SetMsgStep := 1;
   		ELSE
   			COUNTER_WRITE := COUNTER_WRITE + 1;
   		END_IF;
   	9:
   		IF i1030_DI_polarity_w <> i1030_DI_polarity_r
   		THEN
   			LD_OUT := i1030_DI_polarity_w;
   			SetMsg.REQ_LEN := 1;
   			SetMsg.Instance := 1030;
   			SetMsgStep := 1;
   		ELSE
   			COUNTER_WRITE := COUNTER_WRITE + 1;
   		END_IF;
   	10:
   		IF i1537_Controller_parameter_P_w <> i1537_Controller_parameter_P_r
   		THEN
   			LD_OUT := i1537_Controller_parameter_P_w;
   			SetMsg.REQ_LEN := 2;
   			SetMsg.Instance := 1537;
   			SetMsgStep := 1;
   		ELSE
   			COUNTER_WRITE := COUNTER_WRITE + 1;
   		END_IF;
   	11:
   		IF i1538_Controller_parameter_I_w <> i1538_Controller_parameter_I_r
   		THEN
   			LD_OUT := i1538_Controller_parameter_I_w;
   			SetMsg.REQ_LEN := 2;
   			SetMsg.Instance := 1538;
   			SetMsgStep := 1;
   		ELSE
   			COUNTER_WRITE := COUNTER_WRITE + 1;
   		END_IF;
   	12:
   		IF i1539_Controller_parameter_D_w <> i1539_Controller_parameter_D_r
   		THEN
   			LD_OUT := i1539_Controller_parameter_D_w;
   			SetMsg.REQ_LEN := 2;
   			SetMsg.Instance := 1539;
   			SetMsgStep := 1;
   		ELSE
   			COUNTER_WRITE := COUNTER_WRITE + 1;
   		END_IF;
   	13:
   		IF i1540_a_Pos_w <> i1540_a_Pos_r
   		THEN
   			LD_OUT := i1540_a_Pos_w;
   			SetMsg.REQ_LEN := 2;
   			SetMsg.Instance := 1540;
   			SetMsgStep := 1;
   		ELSE
   			COUNTER_WRITE := COUNTER_WRITE + 1;
   		END_IF;
   	14:
   		IF i1541_v_Pos_w <> i1541_v_Pos_r
   		THEN
   			LD_OUT := i1541_v_Pos_w;
   			SetMsg.REQ_LEN := 2;
   			SetMsg.Instance := 1541;
   			SetMsgStep := 1;
   		ELSE
   			COUNTER_WRITE := COUNTER_WRITE + 1;
   		END_IF;
   	15:
   		IF i1542_d_Pos_w <> i1542_d_Pos_r
   		THEN
   			LD_OUT := i1542_d_Pos_w;
   			SetMsg.REQ_LEN := 2;
   			SetMsg.Instance := 1542;
   			SetMsgStep := 1;
   		ELSE
   			COUNTER_WRITE := COUNTER_WRITE + 1;
   		END_IF;
   	16:
   		IF i1543_a_Rot_w <> i1543_a_Rot_r
   		THEN
   			LD_OUT := i1543_a_Rot_w;
   			SetMsg.REQ_LEN := 2;
   			SetMsg.Instance := 1543;
   			SetMsgStep := 1;
   		ELSE
   			COUNTER_WRITE := COUNTER_WRITE + 1;
   		END_IF;
   	17:
   		IF i1544_a_Inch_w <> i1544_a_Inch_r
   		THEN
   			LD_OUT := i1544_a_Inch_w;
   			SetMsg.REQ_LEN := 2;
   			SetMsg.Instance := 1544;
   			SetMsgStep := 1;
   		ELSE
   			COUNTER_WRITE := COUNTER_WRITE + 1;
   		END_IF;
   	18:
   		IF i1545_v_Inch_w <> i1545_v_Inch_r
   		THEN
   			LD_OUT := i1545_v_Inch_w;
   			SetMsg.REQ_LEN := 2;
   			SetMsg.Instance := 1545;
   			SetMsgStep := 1;
   		ELSE
   			COUNTER_WRITE := COUNTER_WRITE + 1;
   		END_IF;
   	19:
   		IF i1546_Pos_window_w <> i1546_Pos_window_r
   		THEN
   			LD_OUT := i1546_Pos_window_w;
   			SetMsg.REQ_LEN := 2;
   			SetMsg.Instance := 1546;
   			SetMsgStep := 1;
   		ELSE
   			COUNTER_WRITE := COUNTER_WRITE + 1;
   		END_IF;
   	20:
   		IF i1547_Gear_ratio_numerator_w <> i1547_Gear_ratio_numerator_r
   		THEN
   			LD_OUT := i1547_Gear_ratio_numerator_w;
   			SetMsg.REQ_LEN := 2;
   			SetMsg.Instance := 1547;
   			SetMsgStep := 1;
   		ELSE
   			COUNTER_WRITE := COUNTER_WRITE + 1;
   		END_IF;
   	21:
   		IF i1548_Gear_ratio_denominator_w <> i1548_Gear_ratio_denominator_r
   		THEN
   			LD_OUT := i1548_Gear_ratio_denominator_w;
   			SetMsg.REQ_LEN := 2;
   			SetMsg.Instance := 1548;
   			SetMsgStep := 1;
   		ELSE
   			COUNTER_WRITE := COUNTER_WRITE + 1;
   		END_IF;
   	22:
   		IF i1549_Spindle_pitch_w <> i1549_Spindle_pitch_r
   		THEN
   			LD_OUT := i1549_Spindle_pitch_w;
   			SetMsg.REQ_LEN := 4;
   			SetMsg.Instance := 1549;
   			SetMsgStep := 1;
   		ELSE
   			COUNTER_WRITE := COUNTER_WRITE + 1;
   		END_IF;
   	23:
   		IF i1550_Calibration_value_w <> i1550_Calibration_value_r
   		THEN
   			LD_OUT := i1550_Calibration_value_w;
   			SetMsg.REQ_LEN := 4;
   			SetMsg.Instance := 1550;
   			SetMsgStep := 1;
   		ELSE
   			COUNTER_WRITE := COUNTER_WRITE + 1;
   		END_IF;
   	24:
   		IF i1551_Limit_1_w <> i1551_Limit_1_r
   		THEN
   			LD_OUT := i1551_Limit_1_w;
   			SetMsg.REQ_LEN := 4;
   			SetMsg.Instance := 1551;
   			SetMsgStep := 1;
   		ELSE
   			COUNTER_WRITE := COUNTER_WRITE + 1;
   		END_IF;
   	25:
   		IF i1552_Limit_2_w <> i1552_Limit_2_r
   		THEN
   			LD_OUT := i1552_Limit_2_w;
   			SetMsg.REQ_LEN := 4;
   			SetMsg.Instance := 1552;
   			SetMsgStep := 1;
   		ELSE
   			COUNTER_WRITE := COUNTER_WRITE + 1;
   		END_IF;
   	26:
   		IF i1553_Delta_inch_w <> i1553_Delta_inch_r
   		THEN
   			LD_OUT := i1553_Delta_inch_w;
   			SetMsg.REQ_LEN := 4;
   			SetMsg.Instance := 1553;
   			SetMsgStep := 1;
   		ELSE
   			COUNTER_WRITE := COUNTER_WRITE + 1;
   		END_IF;
   	27:
   		IF i1554_Sense_of_rotation_w <> i1554_Sense_of_rotation_r
   		THEN
   			LD_OUT := i1554_Sense_of_rotation_w;
   			SetMsg.REQ_LEN := 1;
   			SetMsg.Instance := 1554;
   			SetMsgStep := 1;
   		ELSE
   			COUNTER_WRITE := COUNTER_WRITE + 1;
   		END_IF;
   	28:
   		IF i1555_Pos_type_w <> i1555_Pos_type_r
   		THEN
   			LD_OUT := i1555_Pos_type_w;
   			SetMsg.REQ_LEN := 1;
   			SetMsg.Instance := 1555;
   			SetMsgStep := 1;
   		ELSE
   			COUNTER_WRITE := COUNTER_WRITE + 1;
   		END_IF;
   	29:
   		IF i1556_Operating_mode_w <> i1556_Operating_mode_r
   		THEN
   			LD_OUT := i1556_Operating_mode_w;
   			SetMsg.REQ_LEN := 1;
   			SetMsg.Instance := 1556;
   			SetMsgStep := 1;
   		ELSE
   			COUNTER_WRITE := COUNTER_WRITE + 1;
   		END_IF;
   	30:
   		IF i1557_Inching_2_stop_mode_w <> i1557_Inching_2_stop_mode_r
   		THEN
   			LD_OUT := i1557_Inching_2_stop_mode_w;
   			SetMsg.REQ_LEN := 1;
   			SetMsg.Instance := 1557;
   			SetMsgStep := 1;
   		ELSE
   			COUNTER_WRITE := COUNTER_WRITE + 1;
   		END_IF;
   	31:
   		IF i1558_Inpos_mode_w <> i1558_Inpos_mode_r
   		THEN
   			LD_OUT := i1558_Inpos_mode_w;
   			SetMsg.REQ_LEN := 1;
   			SetMsg.Instance := 1558;
   			SetMsgStep := 1;
   		ELSE
   			COUNTER_WRITE := COUNTER_WRITE + 1;
   		END_IF;
   	32:
   		IF i1559_Loop_length_w <> i1559_Loop_length_r
   		THEN
   			LD_OUT := i1559_Loop_length_w;
   			SetMsg.REQ_LEN := 2;
   			SetMsg.Instance := 1559;
   			SetMsgStep := 1;
   		ELSE
   			COUNTER_WRITE := COUNTER_WRITE + 1;
   		END_IF;
   	33:
   		IF i1560_Contouring_error_limit_w <> i1560_Contouring_error_limit_r
   		THEN
   			LD_OUT := i1560_Contouring_error_limit_w;
   			SetMsg.REQ_LEN := 2;
   			SetMsg.Instance := 1560;
   			SetMsgStep := 1;
   		ELSE
   			COUNTER_WRITE := COUNTER_WRITE + 1;
   		END_IF;
   	34:
   		IF i1561_Current_limiting_w <> i1561_Current_limiting_r
   		THEN
   			LD_OUT := i1561_Current_limiting_w;
   			SetMsg.REQ_LEN := 1;
   			SetMsg.Instance := 1561;
   			SetMsgStep := 1;
   		ELSE
   			COUNTER_WRITE := COUNTER_WRITE + 1;
   		END_IF;
   	35:
   		IF i1562_Inching_2_Offset_w <> i1562_Inching_2_Offset_r
   		THEN
   			LD_OUT := i1562_Inching_2_Offset_w;
   			SetMsg.REQ_LEN := 1;
   			SetMsg.Instance := 1562;
   			SetMsgStep := 1;
   		ELSE
   			COUNTER_WRITE := COUNTER_WRITE + 1;
   		END_IF;
   	36:
   		IF i1563_Inching_2_acceleration_type_w <> i1563_Inching_2_acceleration_type_r
   		THEN
   			LD_OUT := i1563_Inching_2_acceleration_type_w;
   			SetMsg.REQ_LEN := 1;
   			SetMsg.Instance := 1563;
   			SetMsgStep := 1;
   		ELSE
   			COUNTER_WRITE := COUNTER_WRITE + 1;
   		END_IF;
   	37:
   		IF i1564_Offset_w <> i1564_Offset_r
   		THEN
   			LD_OUT := i1564_Offset_w;
   			SetMsg.REQ_LEN := 4;
   			SetMsg.Instance := 1564;
   			SetMsgStep := 1;
   		ELSE
   			COUNTER_WRITE := COUNTER_WRITE + 1;
   		END_IF;
   	38:
   		IF i2338_Pcm_pos_1_w <> i2338_Pcm_pos_1_r
   		THEN
   			LD_OUT := i2338_Pcm_pos_1_w;
   			SetMsg.REQ_LEN := 4;
   			SetMsg.Instance := 2338;
   			SetMsgStep := 1;
   		ELSE
   			COUNTER_WRITE := COUNTER_WRITE + 1;
   		END_IF;
   	39:
   		IF i2339_Pcm_pos_2_w <> i2339_Pcm_pos_2_r
   		THEN
   			LD_OUT := i2339_Pcm_pos_2_w;
   			SetMsg.REQ_LEN := 4;
   			SetMsg.Instance := 2339;
   			SetMsgStep := 1;
   		ELSE
   			COUNTER_WRITE := COUNTER_WRITE + 1;
   		END_IF;
   	40:
   		IF i2340_Pcm_pos_3_w <> i2340_Pcm_pos_3_r
   		THEN
   			LD_OUT := i2340_Pcm_pos_3_w;
   			SetMsg.REQ_LEN := 4;
   			SetMsg.Instance := 2340;
   			SetMsgStep := 1;
   		ELSE
   			COUNTER_WRITE := COUNTER_WRITE + 1;
   		END_IF;
   	41:
   		IF i2341_Pcm_pos_4_w <> i2341_Pcm_pos_4_r
   		THEN
   			LD_OUT := i2341_Pcm_pos_4_w;
   			SetMsg.REQ_LEN := 4;
   			SetMsg.Instance := 2341;
   			SetMsgStep := 1;
   		ELSE
   			COUNTER_WRITE := COUNTER_WRITE + 1;
   		END_IF;
   	42:
   		IF i2342_Pcm_pos_5_w <> i2342_Pcm_pos_5_r
   		THEN
   			LD_OUT := i2342_Pcm_pos_5_w;
   			SetMsg.REQ_LEN := 4;
   			SetMsg.Instance := 2342;
   			SetMsgStep := 1;
   		ELSE
   			COUNTER_WRITE := COUNTER_WRITE + 1;
   		END_IF;
   	43:
   		IF i2343_Pcm_pos_6_w <> i2343_Pcm_pos_6_r
   		THEN
   			LD_OUT := i2343_Pcm_pos_6_w;
   			SetMsg.REQ_LEN := 4;
   			SetMsg.Instance := 2343;
   			SetMsgStep := 1;
   		ELSE
   			COUNTER_WRITE := COUNTER_WRITE + 1;
   		END_IF;
   	44:
   		IF i2344_Pcm_pos_7_w <> i2344_Pcm_pos_7_r
   		THEN
   			LD_OUT := i2344_Pcm_pos_7_w;
   			SetMsg.REQ_LEN := 4;
   			SetMsg.Instance := 2344;
   			SetMsgStep := 1;
   		ELSE
   			COUNTER_WRITE := COUNTER_WRITE + 1;
   		END_IF;
   	45:
   		IF i2370_Pcm_acc_1_w <> i2370_Pcm_acc_1_r
   		THEN
   			LD_OUT := i2370_Pcm_acc_1_w;
   			SetMsg.REQ_LEN := 2;
   			SetMsg.Instance := 2370;
   			SetMsgStep := 1;
   		ELSE
   			COUNTER_WRITE := COUNTER_WRITE + 1;
   		END_IF;
   	46:
   		IF i2371_Pcm_acc_2_w <> i2371_Pcm_acc_2_r
   		THEN
   			LD_OUT := i2371_Pcm_acc_2_w;
   			SetMsg.REQ_LEN := 2;
   			SetMsg.Instance := 2371;
   			SetMsgStep := 1;
   		ELSE
   			COUNTER_WRITE := COUNTER_WRITE + 1;
   		END_IF;
   	47:
   		IF i2372_Pcm_acc_3_w <> i2372_Pcm_acc_3_r
   		THEN
   			LD_OUT := i2372_Pcm_acc_3_w;
   			SetMsg.REQ_LEN := 2;
   			SetMsg.Instance := 2372;
   			SetMsgStep := 1;
   		ELSE
   			COUNTER_WRITE := COUNTER_WRITE + 1;
   		END_IF;
   	48:
   		IF i2373_Pcm_acc_4_w <> i2373_Pcm_acc_4_r
   		THEN
   			LD_OUT := i2373_Pcm_acc_4_w;
   			SetMsg.REQ_LEN := 2;
   			SetMsg.Instance := 2373;
   			SetMsgStep := 1;
   		ELSE
   			COUNTER_WRITE := COUNTER_WRITE + 1;
   		END_IF;
   	49:
   		IF i2374_Pcm_acc_5_w <> i2374_Pcm_acc_5_r
   		THEN
   			LD_OUT := i2374_Pcm_acc_5_w;
   			SetMsg.REQ_LEN := 2;
   			SetMsg.Instance := 2374;
   			SetMsgStep := 1;
   		ELSE
   			COUNTER_WRITE := COUNTER_WRITE + 1;
   		END_IF;
   	50:
   		IF i2375_Pcm_acc_6_w <> i2375_Pcm_acc_6_r
   		THEN
   			LD_OUT := i2375_Pcm_acc_6_w;
   			SetMsg.REQ_LEN := 2;
   			SetMsg.Instance := 2375;
   			SetMsgStep := 1;
   		ELSE
   			COUNTER_WRITE := COUNTER_WRITE + 1;
   		END_IF;
   	51:
   		IF i2376_Pcm_acc_7_w <> i2376_Pcm_acc_7_r
   		THEN
   			LD_OUT := i2376_Pcm_acc_7_w;
   			SetMsg.REQ_LEN := 2;
   			SetMsg.Instance := 2376;
   			SetMsgStep := 1;
   		ELSE
   			COUNTER_WRITE := COUNTER_WRITE + 1;
   		END_IF;
   	52:
   		IF i2402_Pcm_vel_1_w <> i2402_Pcm_vel_1_r
   		THEN
   			LD_OUT := i2402_Pcm_vel_1_w;
   			SetMsg.REQ_LEN := 2;
   			SetMsg.Instance := 2402;
   			SetMsgStep := 1;
   		ELSE
   			COUNTER_WRITE := COUNTER_WRITE + 1;
   		END_IF;
   	53:
   		IF i2403_Pcm_vel_2_w <> i2403_Pcm_vel_2_r
   		THEN
   			LD_OUT := i2403_Pcm_vel_2_w;
   			SetMsg.REQ_LEN := 2;
   			SetMsg.Instance := 2403;
   			SetMsgStep := 1;
   		ELSE
   			COUNTER_WRITE := COUNTER_WRITE + 1;
   		END_IF;
   	54:
   		IF i2404_Pcm_vel_3_w <> i2404_Pcm_vel_3_r
   		THEN
   			LD_OUT := i2404_Pcm_vel_3_w;
   			SetMsg.REQ_LEN := 2;
   			SetMsg.Instance := 2404;
   			SetMsgStep := 1;
   		ELSE
   			COUNTER_WRITE := COUNTER_WRITE + 1;
   		END_IF;
   	55:
   		IF i2405_Pcm_vel_4_w <> i2405_Pcm_vel_4_r
   		THEN
   			LD_OUT := i2405_Pcm_vel_4_w;
   			SetMsg.REQ_LEN := 2;
   			SetMsg.Instance := 2405;
   			SetMsgStep := 1;
   		ELSE
   			COUNTER_WRITE := COUNTER_WRITE + 1;
   		END_IF;
   	56:
   		IF i2406_Pcm_vel_5_w <> i2406_Pcm_vel_5_r
   		THEN
   			LD_OUT := i2406_Pcm_vel_5_w;
   			SetMsg.REQ_LEN := 2;
   			SetMsg.Instance := 2406;
   			SetMsgStep := 1;
   		ELSE
   			COUNTER_WRITE := COUNTER_WRITE + 1;
   		END_IF;
   	57:
   		IF i2407_Pcm_vel_6_w <> i2407_Pcm_vel_6_r
   		THEN
   			LD_OUT := i2407_Pcm_vel_6_w;
   			SetMsg.REQ_LEN := 2;
   			SetMsg.Instance := 2407;
   			SetMsgStep := 1;
   		ELSE
   			COUNTER_WRITE := COUNTER_WRITE + 1;
   		END_IF;
   	58:
   		IF i2408_Pcm_vel_7_w <> i2408_Pcm_vel_7_r
   		THEN
   			LD_OUT := i2408_Pcm_vel_7_w;
   			SetMsg.REQ_LEN := 2;
   			SetMsg.Instance := 2408;
   			SetMsgStep := 1;
   		ELSE
   			COUNTER_WRITE := COUNTER_WRITE + 1;
   		END_IF;
   	59:
   		IF i2434_Pcm_dec_1_w <> i2434_Pcm_dec_1_r
   		THEN
   			LD_OUT := i2434_Pcm_dec_1_w;
   			SetMsg.REQ_LEN := 2;
   			SetMsg.Instance := 2434;
   			SetMsgStep := 1;
   		ELSE
   			COUNTER_WRITE := COUNTER_WRITE + 1;
   		END_IF;
   	60:
   		IF i2435_Pcm_dec_2_w <> i2435_Pcm_dec_2_r
   		THEN
   			LD_OUT := i2435_Pcm_dec_2_w;
   			SetMsg.REQ_LEN := 2;
   			SetMsg.Instance := 2435;
   			SetMsgStep := 1;
   		ELSE
   			COUNTER_WRITE := COUNTER_WRITE + 1;
   		END_IF;
   	61:
   		IF i2436_Pcm_dec_3_w <> i2436_Pcm_dec_3_r
   		THEN
   			LD_OUT := i2436_Pcm_dec_3_w;
   			SetMsg.REQ_LEN := 2;
   			SetMsg.Instance := 2436;
   			SetMsgStep := 1;
   		ELSE
   			COUNTER_WRITE := COUNTER_WRITE + 1;
   		END_IF;
   	62:
   		IF i2437_Pcm_dec_4_w <> i2437_Pcm_dec_4_r
   		THEN
   			LD_OUT := i2437_Pcm_dec_4_w;
   			SetMsg.REQ_LEN := 2;
   			SetMsg.Instance := 2437;
   			SetMsgStep := 1;
   		ELSE
   			COUNTER_WRITE := COUNTER_WRITE + 1;
   		END_IF;
   	63:
   		IF i2438_Pcm_dec_5_w <> i2438_Pcm_dec_5_r
   		THEN
   			LD_OUT := i2438_Pcm_dec_5_w;
   			SetMsg.REQ_LEN := 2;
   			SetMsg.Instance := 2438;
   			SetMsgStep := 1;
   		ELSE
   			COUNTER_WRITE := COUNTER_WRITE + 1;
   		END_IF;
   	64:
   		IF i2439_Pcm_dec_6_w <> i2439_Pcm_dec_6_r
   		THEN
   			LD_OUT := i2439_Pcm_dec_6_w;
   			SetMsg.REQ_LEN := 2;
   			SetMsg.Instance := 2439;
   			SetMsgStep := 1;
   		ELSE
   			COUNTER_WRITE := COUNTER_WRITE + 1;
   		END_IF;
   	65:
   		IF i2440_Pcm_dec_7_w <> i2440_Pcm_dec_7_r
   		THEN
   			LD_OUT := i2440_Pcm_dec_7_w;
   			SetMsg.REQ_LEN := 2;
   			SetMsg.Instance := 2440;
   			SetMsgStep := 1;
   		ELSE
   			COUNTER_WRITE := COUNTER_WRITE + 1;
   		END_IF;
   	66:
   		IF i3073_S_command_w <> i3073_S_command_r
   		THEN
   			LD_OUT := i3073_S_command_w;
   			SetMsg.REQ_LEN := 1;
   			SetMsg.Instance := 3073;
   			SetMsgStep := 1;
   		ELSE
   			COUNTER_WRITE := COUNTER_WRITE + 1;
   		END_IF;
   	END_CASE;
   	// output count_write value
   	count_write := COUNTER_WRITE;
   END_IF;
   
   // send message
   IF (SetMsgStep = 1) THEN
   	// DINT TO SINT[4]
   	COP(LD_OUT,SetMsgData[0],4);
   
   	MSG(SetMsg);
   
   	SetMsgStep := 2;
   END_IF;
   
   // create local copy of WriteTag.FLAGS
   SetMsgFlags := SetMsg.FLAGS;
   
   IF(SetMsgStep = 2) AND (SetMsgFlags.4) THEN
   // .ER bit set = transfer failed
    	SetMsgStep := 0;
   	write_error := 0;
   
   	// copy error code to write_error
   	BTDT_02.Source := SetMsg.ERR;
   	BTDT_02.SourceBit := 0;
   	BTDT_02.Length := 16;
   	BTDT_02.DestBit := 0;
   	BTDT_02.Target := write_error;
   	BTDT(BTDT_02);
   	write_error := BTDT_02.Dest;
   
   	// copy extended error code to write_error
   	BTDT_02.Source := SetMsg.EXERR;
   	BTDT_02.SourceBit := 0;
   	BTDT_02.Length := 16;
   	BTDT_02.DestBit := 16;
   	BTDT_02.Target := write_error;
   	BTDT(BTDT_02);
   	write_error := BTDT_02.Dest;
   
   	// set status bits
   	Sts_Done := 0;
   	Sts_Busy := 0;
   	Sts_General_error := 1;
   
   	COUNTER_WRITE := 0;
   
   ELSIF (SetMsgStep = 2) AND (SetMsgFlags.5) THEN
   // .DN bit set = transfer ok
   	SetMsgStep := 0;
   	write_error := 0;
   
   
   	CASE COUNTER_WRITE OF // write response
   	1:
   		i0513_Led_functionality_r := i0513_Led_functionality_w;
   	2:
   		i0545_Si_baudrate_r := i0545_Si_baudrate_w;
   	3:
   		i0769_DO_1_functionality_r := i0769_DO_1_functionality_w;
   	4:
   		i0771_DO_polarity_r := i0771_DO_polarity_w;
   	5:
   		i1025_DI_1_functionality_r := i1025_DI_1_functionality_w;
   	6:
   		i1026_DI_2_functionality_r := i1026_DI_2_functionality_w;
   	7:
   		i1027_DI_3_functionality_r := i1027_DI_3_functionality_w;
   	8:
   		i1028_DI_4_functionality_r := i1028_DI_4_functionality_w;
   	9:
   		i1030_DI_polarity_r := i1030_DI_polarity_w;
   	10:
   		i1537_Controller_parameter_P_r := i1537_Controller_parameter_P_w;
   	11:
   		i1538_Controller_parameter_I_r := i1538_Controller_parameter_I_w;
   	12:
   		i1539_Controller_parameter_D_r := i1539_Controller_parameter_D_w;
   	13:
   		i1540_a_Pos_r := i1540_a_Pos_w;
   	14:
   		i1541_v_Pos_r := i1541_v_Pos_w;
   	15:
   		i1542_d_Pos_r := i1542_d_Pos_w;
   	16:
   		i1543_a_Rot_r := i1543_a_Rot_w;
   	17:
   		i1544_a_Inch_r := i1544_a_Inch_w;
   	18:
   		i1545_v_Inch_r := i1545_v_Inch_w;
   	19:
   		i1546_Pos_window_r := i1546_Pos_window_w;
   	20:
   		i1547_Gear_ratio_numerator_r := i1547_Gear_ratio_numerator_w;
   	21:
   		i1548_Gear_ratio_denominator_r := i1548_Gear_ratio_denominator_w;
   	22:
   		i1549_Spindle_pitch_r := i1549_Spindle_pitch_w;
   	23:
   		i1550_Calibration_value_r := i1550_Calibration_value_w;
   	24:
   		i1551_Limit_1_r := i1551_Limit_1_w;
   	25:
   		i1552_Limit_2_r := i1552_Limit_2_w;
   	26:
   		i1553_Delta_inch_r := i1553_Delta_inch_w;
   	27:
   		i1554_Sense_of_rotation_r := i1554_Sense_of_rotation_w;
   	28:
   		i1555_Pos_type_r := i1555_Pos_type_w;
   	29:
   		i1556_Operating_mode_r := i1556_Operating_mode_w;
   	30:
   		i1557_Inching_2_stop_mode_r := i1557_Inching_2_stop_mode_w;
   	31:
   		i1558_Inpos_mode_r := i1558_Inpos_mode_w;
   	32:
   		i1559_Loop_length_r := i1559_Loop_length_w;
   	33:
   		i1560_Contouring_error_limit_r := i1560_Contouring_error_limit_w;
   	34:
   		i1561_Current_limiting_r := i1561_Current_limiting_w;
   	35:
   		i1562_Inching_2_Offset_r := i1562_Inching_2_Offset_w;
   	36:
   		i1563_Inching_2_acceleration_type_r := i1563_Inching_2_acceleration_type_w;
   	37:
   		i1564_Offset_r := i1564_Offset_w;
   	38:
   		i2338_Pcm_pos_1_r := i2338_Pcm_pos_1_w;
   	39:
   		i2339_Pcm_pos_2_r := i2339_Pcm_pos_2_w;
   	40:
   		i2340_Pcm_pos_3_r := i2340_Pcm_pos_3_w;
   	41:
   		i2341_Pcm_pos_4_r := i2341_Pcm_pos_4_w;
   	42:
   		i2342_Pcm_pos_5_r := i2342_Pcm_pos_5_w;
   	43:
   		i2343_Pcm_pos_6_r := i2343_Pcm_pos_6_w;
   	44:
   		i2344_Pcm_pos_7_r := i2344_Pcm_pos_7_w;
   	45:
   		i2370_Pcm_acc_1_r := i2370_Pcm_acc_1_w;
   	46:
   		i2371_Pcm_acc_2_r := i2371_Pcm_acc_2_w;
   	47:
   		i2372_Pcm_acc_3_r := i2372_Pcm_acc_3_w;
   	48:
   		i2373_Pcm_acc_4_r := i2373_Pcm_acc_4_w;
   	49:
   		i2374_Pcm_acc_5_r := i2374_Pcm_acc_5_w;
   	50:
   		i2375_Pcm_acc_6_r := i2375_Pcm_acc_6_w;
   	51:
   		i2376_Pcm_acc_7_r := i2376_Pcm_acc_7_w;
   	52:
   		i2402_Pcm_vel_1_r := i2402_Pcm_vel_1_w;
   	53:
   		i2403_Pcm_vel_2_r := i2403_Pcm_vel_2_w;
   	54:
   		i2404_Pcm_vel_3_r := i2404_Pcm_vel_3_w;
   	55:
   		i2405_Pcm_vel_4_r := i2405_Pcm_vel_4_w;
   	56:
   		i2406_Pcm_vel_5_r := i2406_Pcm_vel_5_w;
   	57:
   		i2407_Pcm_vel_6_r := i2407_Pcm_vel_6_w;
   	58:
   		i2408_Pcm_vel_7_r := i2408_Pcm_vel_7_w;
   	59:
   		i2434_Pcm_dec_1_r := i2434_Pcm_dec_1_w;
   	60:
   		i2435_Pcm_dec_2_r := i2435_Pcm_dec_2_w;
   	61:
   		i2436_Pcm_dec_3_r := i2436_Pcm_dec_3_w;
   	62:
   		i2437_Pcm_dec_4_r := i2437_Pcm_dec_4_w;
   	63:
   		i2438_Pcm_dec_5_r := i2438_Pcm_dec_5_w;
   	64:
   		i2439_Pcm_dec_6_r := i2439_Pcm_dec_6_w;
   	65:
   		i2440_Pcm_dec_7_r := i2440_Pcm_dec_7_w;
   	66:
       	i3073_S_command_r := 0; // set always to zero
   	END_CASE;
   	COUNTER_WRITE := COUNTER_WRITE + 1;
   END_IF;
   
   IF (COUNTER_WRITE > 66)
   THEN
   	COUNTER_WRITE := 0;
   	count_write := COUNTER_WRITE;
   
   	// set status bits
   	Sts_Done := 1;
   	Sts_Busy := 0;
   	Sts_General_error := 0;
   
   END_IF;
   
   ///////////////////////////////////////////////////////////////////////////////////////////////
   // handle copy instruction
   //
   
   IF (COUNTER_COPY > 0)
   THEN
   	i0513_Led_functionality_w := i0513_Led_functionality_r;
   	i0545_Si_baudrate_w := i0545_Si_baudrate_r;
   	i0769_DO_1_functionality_w := i0769_DO_1_functionality_r;
   	i0771_DO_polarity_w := i0771_DO_polarity_r;
   	i1025_DI_1_functionality_w := i1025_DI_1_functionality_r;
   	i1026_DI_2_functionality_w := i1026_DI_2_functionality_r;
   	i1027_DI_3_functionality_w := i1027_DI_3_functionality_r;
   	i1028_DI_4_functionality_w := i1028_DI_4_functionality_r;
   	i1030_DI_polarity_w := i1030_DI_polarity_r;
   	i1537_Controller_parameter_P_w := i1537_Controller_parameter_P_r;
   	i1538_Controller_parameter_I_w := i1538_Controller_parameter_I_r;
   	i1539_Controller_parameter_D_w := i1539_Controller_parameter_D_r;
   	i1540_a_Pos_w := i1540_a_Pos_r;
   	i1541_v_Pos_w := i1541_v_Pos_r;
   	i1542_d_Pos_w := i1542_d_Pos_r;
   	i1543_a_Rot_w := i1543_a_Rot_r;
   	i1544_a_Inch_w := i1544_a_Inch_r;
   	i1545_v_Inch_w := i1545_v_Inch_r;
   	i1546_Pos_window_w := i1546_Pos_window_r;
   	i1547_Gear_ratio_numerator_w := i1547_Gear_ratio_numerator_r;
   	i1548_Gear_ratio_denominator_w := i1548_Gear_ratio_denominator_r;
   	i1549_Spindle_pitch_w := i1549_Spindle_pitch_r;
   	i1550_Calibration_value_w := i1550_Calibration_value_r;
   	i1551_Limit_1_w := i1551_Limit_1_r;
   	i1552_Limit_2_w := i1552_Limit_2_r;
   	i1553_Delta_inch_w := i1553_Delta_inch_r;
   	i1554_Sense_of_rotation_w := i1554_Sense_of_rotation_r;
   	i1555_Pos_type_w := i1555_Pos_type_r;
   	i1556_Operating_mode_w := i1556_Operating_mode_r;
   	i1557_Inching_2_stop_mode_w := i1557_Inching_2_stop_mode_r;
   	i1558_Inpos_mode_w := i1558_Inpos_mode_r;
   	i1559_Loop_length_w := i1559_Loop_length_r;
   	i1560_Contouring_error_limit_w := i1560_Contouring_error_limit_r;
   	i1561_Current_limiting_w := i1561_Current_limiting_r;
   	i1562_Inching_2_Offset_w := i1562_Inching_2_Offset_r;
   	i1563_Inching_2_acceleration_type_w := i1563_Inching_2_acceleration_type_r;
   	i1564_Offset_w := i1564_Offset_r;
   	i2338_Pcm_pos_1_w := i2338_Pcm_pos_1_r;
   	i2339_Pcm_pos_2_w := i2339_Pcm_pos_2_r;
   	i2340_Pcm_pos_3_w := i2340_Pcm_pos_3_r;
   	i2341_Pcm_pos_4_w := i2341_Pcm_pos_4_r;
   	i2342_Pcm_pos_5_w := i2342_Pcm_pos_5_r;
   	i2343_Pcm_pos_6_w := i2343_Pcm_pos_6_r;
   	i2344_Pcm_pos_7_w := i2344_Pcm_pos_7_r;
   	i2370_Pcm_acc_1_w := i2370_Pcm_acc_1_r;
   	i2371_Pcm_acc_2_w := i2371_Pcm_acc_2_r;
   	i2372_Pcm_acc_3_w := i2372_Pcm_acc_3_r;
   	i2373_Pcm_acc_4_w := i2373_Pcm_acc_4_r;
   	i2374_Pcm_acc_5_w := i2374_Pcm_acc_5_r;
   	i2375_Pcm_acc_6_w := i2375_Pcm_acc_6_r;
   	i2376_Pcm_acc_7_w := i2376_Pcm_acc_7_r;
   	i2402_Pcm_vel_1_w := i2402_Pcm_vel_1_r;
   	i2403_Pcm_vel_2_w := i2403_Pcm_vel_2_r;
   	i2404_Pcm_vel_3_w := i2404_Pcm_vel_3_r;
   	i2405_Pcm_vel_4_w := i2405_Pcm_vel_4_r;
   	i2406_Pcm_vel_5_w := i2406_Pcm_vel_5_r;
   	i2407_Pcm_vel_6_w := i2407_Pcm_vel_6_r;
   	i2408_Pcm_vel_7_w := i2408_Pcm_vel_7_r;
   	i2434_Pcm_dec_1_w := i2434_Pcm_dec_1_r;
   	i2435_Pcm_dec_2_w := i2435_Pcm_dec_2_r;
   	i2436_Pcm_dec_3_w := i2436_Pcm_dec_3_r;
   	i2437_Pcm_dec_4_w := i2437_Pcm_dec_4_r;
   	i2438_Pcm_dec_5_w := i2438_Pcm_dec_5_r;
   	i2439_Pcm_dec_6_w := i2439_Pcm_dec_6_r;
   	i2440_Pcm_dec_7_w := i2440_Pcm_dec_7_r;
   
   	COUNTER_COPY := COUNTER_COPY + 1;
   END_IF;
   
   IF (COUNTER_COPY > 1)
   THEN
   	COUNTER_COPY := 0;
   
   	// set status bits
   	Sts_Done := 1;
   	Sts_Busy := 0;
   	Sts_General_error := 0;
   
   END_IF;
   
   ///////////////////////////////////////////////////////////////////////////////////////////////
   // actual value
   // SINT[4] TO DIND
   
   COP (DC_INPUT_BUF[2],ACTUAL_VALUE,1);
   
   ///////////////////////////////////////////////////////////////////////////////////////////////
   // status word
   //
   
   Sts_Supply 					:= DC_INPUT_BUF[0].0;
   Sts_Readiness_to_travel 	:= DC_INPUT_BUF[0].1;
   Sts_Upper_limit 			:= DC_INPUT_BUF[0].2;
   Sts_Lower_limit 			:= DC_INPUT_BUF[0].3;
   Sts_Actuator_travels_stands := DC_INPUT_BUF[0].4;
   Sts_InPos 					:= DC_INPUT_BUF[0].5;
   Sts_Active_travel_job 		:= DC_INPUT_BUF[0].6;
   Sts_Error 					:= DC_INPUT_BUF[0].7;
   Sts_Operation_enabled 		:= DC_INPUT_BUF[1].0;
   Sts_Switch_lock 			:= DC_INPUT_BUF[1].1;
   Sts_Travel_job_acknowledge 	:= DC_INPUT_BUF[1].2;
   Sts_Battery_warning 		:= DC_INPUT_BUF[1].3;
   Sts_Current_limiting 		:= DC_INPUT_BUF[1].4;
   Sts_BIT13 					:= DC_INPUT_BUF[1].5;
   Sts_BIT14 					:= DC_INPUT_BUF[1].6;
   Sts_BIT15 					:= DC_INPUT_BUF[1].7;
   
   ///////////////////////////////////////////////////////////////////////////////////////////////
   // digital inputs
   //
   Sts_DI1 					:= DC_INPUT_BUF[6].0;
   Sts_DI2 					:= DC_INPUT_BUF[6].1;
   Sts_DI3	 					:= DC_INPUT_BUF[6].2;
   Sts_DI4 					:= DC_INPUT_BUF[6].3;
   
   ///////////////////////////////////////////////////////////////////////////////////////////////
   // write outputs synchonous
   
   CPS(DC_OUTPUT_BUF[0],DC_OUTPUT[0],7);
END_ROUTINE
END_ADD_ON_INSTRUCTION
